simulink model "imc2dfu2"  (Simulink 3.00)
settings: Solver=ode45  SolverMode=SingleTasking  StartTime=0.0  StopTime=10  FixedStep=st_size  MaxStep=st_size  RelTol=1e-5  AbsTol=1e-6
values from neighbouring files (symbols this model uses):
  Disturb = Setpoint    [mimo_MSF1DF_sim.m]    (also in mimo_MSF2DF_sim.m)
  Satlb = temp1    [cback.m]    (also in imcmenu.m = str2num(satlbs))
  Satub = temp1    [cback.m]    (also in imcmenu.m = str2num(satubs))
  Setpoint = zeros(1,n)    [mimo_MSF1DF_sim.m]    (also in mimo_MSF2DF_sim.m)
undefined symbols (not defined in the file or in its folder): Csden, Csnum, pdeadx, Pre_fil_den, Pre_fil_num, XdenPs, XnumPs

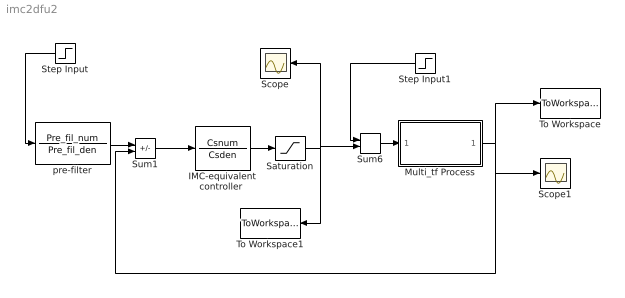
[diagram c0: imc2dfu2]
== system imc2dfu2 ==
  "IMC-equivalent controller " : TransferFcn  Numerator=Csnum  Denominator=Csden
  Multi_tf Process : Subsystem
  Saturation : Saturate  UpperLimit=Satub  LowerLimit=Satlb
  Scope : Scope
  Scope1 : Scope
  Step Input : Step  Orientation=left  Time=0  Before=0  After=Setpoint  SampleTime=0
  Step Input1 : Step  Orientation=left  Time=0  Before=0  After=Disturb  SampleTime=0
  Sum1 : Sum  Inputs=+-  SaturateOnIntegerOverflow=on
  Sum6 : Sum  Inputs=++  SaturateOnIntegerOverflow=on
  To Workspace : ToWorkspace  VariableName=simout  SampleTime=-1  SaveFormat=Matrix
  To Workspace1 : ToWorkspace  VariableName=effort  SampleTime=-1  SaveFormat=Matrix
  pre-filter : TransferFcn  Numerator=Pre_fil_num  Denominator=Pre_fil_den
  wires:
  Sum1/1 -> "IMC-equivalent controller "/1
  Step Input/1 -> pre-filter/1
  "IMC-equivalent controller "/1 -> Saturation/1
  pre-filter/1 -> Sum1/1
  Step Input1/1 -> Sum6/1
  Saturation/1 -> Sum6/2, Scope/1, To Workspace1/1
  Sum6/1 -> Multi_tf Process/1(In1)
  Multi_tf Process/1(Out1) -> Sum1/2, To Workspace/1, Scope1/1

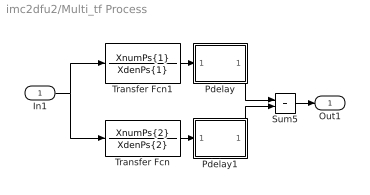
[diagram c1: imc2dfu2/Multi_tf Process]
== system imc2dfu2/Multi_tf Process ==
  In1 : Inport  Port=1  PortWidth=-1  SampleTime=-1  DataType=auto
  Pdelay : Subsystem
  Pdelay1 : Subsystem
  Sum5 : Sum  Inputs=++  SaturateOnIntegerOverflow=on
  Transfer Fcn : TransferFcn  Numerator=XnumPs{2}  Denominator=XdenPs{2}
  Transfer Fcn1 : TransferFcn  Numerator=XnumPs{1}  Denominator=XdenPs{1}
  Out1 : Outport  Port=1  InitialOutput=0
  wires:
  Transfer Fcn1/1 -> Pdelay/1(In1)
  Transfer Fcn/1 -> Pdelay1/1(In1)
  In1/1 -> Transfer Fcn1/1, Transfer Fcn/1
  Sum5/1 -> Out1/1
  Pdelay/1(Out1) -> Sum5/1
  Pdelay1/1(Out1) -> Sum5/2

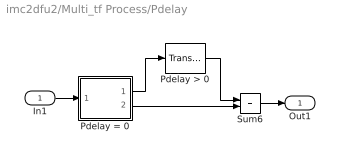
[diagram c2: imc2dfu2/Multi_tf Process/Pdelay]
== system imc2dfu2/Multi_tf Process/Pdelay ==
  In1 : Inport  Port=1  PortWidth=-1  SampleTime=-1  DataType=auto
  Pdelay > 0 : TransportDelay  DelayTime=pdeadx(1)  InitialInput=0  BufferSize=1024
  Pdelay = 0 : Subsystem  Description=pass input signal through out1 if condition is true.
  Sum6 : Sum  Inputs=++  SaturateOnIntegerOverflow=on
  Out1 : Outport  Port=1
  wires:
  Pdelay = 0/1(Out2) -> Pdelay > 0/1
  Pdelay > 0/1 -> Sum6/1
  Pdelay = 0/2(Out1) -> Sum6/2
  In1/1 -> Pdelay = 0/1(In)
  Sum6/1 -> Out1/1

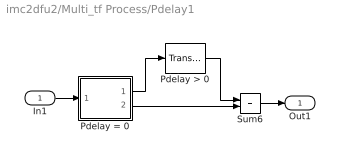
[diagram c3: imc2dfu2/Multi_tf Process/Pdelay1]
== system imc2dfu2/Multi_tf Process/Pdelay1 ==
  In1 : Inport  Port=1  PortWidth=-1  SampleTime=-1  DataType=auto
  Pdelay > 0 : TransportDelay  DelayTime=pdeadx(2)  InitialInput=0  BufferSize=1024
  Pdelay = 0 : Subsystem  Description=pass input signal through out1 if condition is true.
  Sum6 : Sum  Inputs=++  SaturateOnIntegerOverflow=on
  Out1 : Outport  Port=1
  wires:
  Pdelay = 0/1(Out2) -> Pdelay > 0/1
  Pdelay > 0/1 -> Sum6/1
  Pdelay = 0/2(Out1) -> Sum6/2
  In1/1 -> Pdelay = 0/1(In)
  Sum6/1 -> Out1/1

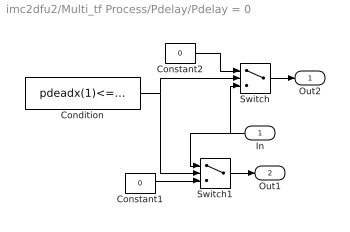
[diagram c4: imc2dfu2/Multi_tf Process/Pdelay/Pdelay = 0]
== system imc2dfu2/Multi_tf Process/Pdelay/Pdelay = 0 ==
  In : Inport  Orientation=left  Port=1  PortWidth=-1  SampleTime=-1  DataType=auto
  Condition : Constant  Value=pdeadx(1)<=3*eps
  Constant1 : Constant  Value=0
  Constant2 : Constant  Value=0
  Switch : Switch  Threshold=1
  Switch1 : Switch  Threshold=1
  Out2 : Outport  Port=1  InitialOutput=0
  Out1 : Outport  Port=2  InitialOutput=0
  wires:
  In/1 -> Switch/3, Switch1/1
  Condition/1 -> Switch1/2, Switch/2
  Constant1/1 -> Switch1/3
  Constant2/1 -> Switch/1
  Switch/1 -> Out2/1
  Switch1/1 -> Out1/1

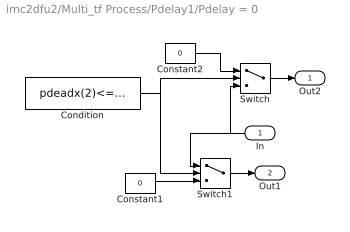
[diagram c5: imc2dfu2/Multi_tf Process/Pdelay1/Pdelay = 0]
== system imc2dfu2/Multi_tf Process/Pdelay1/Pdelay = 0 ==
  In : Inport  Orientation=left  Port=1  PortWidth=-1  SampleTime=-1  DataType=auto
  Condition : Constant  Value=pdeadx(2)<=3*eps
  Constant1 : Constant  Value=0
  Constant2 : Constant  Value=0
  Switch : Switch  Threshold=1
  Switch1 : Switch  Threshold=1
  Out2 : Outport  Port=1  InitialOutput=0
  Out1 : Outport  Port=2  InitialOutput=0
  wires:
  In/1 -> Switch/3, Switch1/1
  Condition/1 -> Switch1/2, Switch/2
  Constant1/1 -> Switch1/3
  Constant2/1 -> Switch/1
  Switch/1 -> Out2/1
  Switch1/1 -> Out1/1
